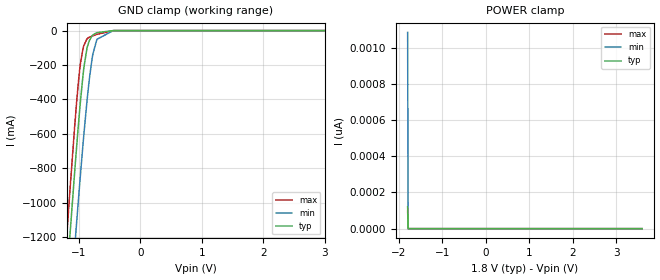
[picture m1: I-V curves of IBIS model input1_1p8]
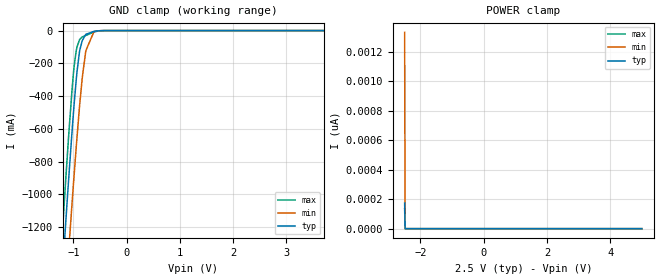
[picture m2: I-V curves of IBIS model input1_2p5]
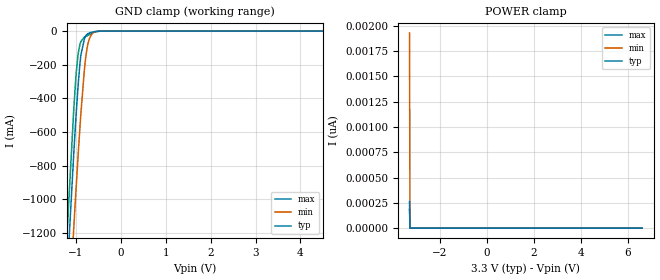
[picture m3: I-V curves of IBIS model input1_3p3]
| Texas Instruments Incorporated
| ADS93xx
| 2-Channel, 16-Bit 5/3 MSPS per channel
[IBIS Ver]   4.1
[File name]   ads93xx.ibs
[File Rev]   1.0
[Date]   28/03/2025
[Source]
| Texas Instruments Incorporated.
| Analog-eLab Design Center, HPA
| 12500 TI Blvd
| Dallas, TX -75243
[Notes]   Revision History:
| Rev 1.0: 28/03/2025
| - Initial version of the model
| - Model generated from simulations in SPECTRE
| - Model matched to SPICE simulation
| - C_comp although listed in numerical order of value are
|   obtained from varying PVT conditions. For PVT conditions for
|   each specific value refer the buffer description under
|   respective [Model]. IBIS model user is responsible for using
|   appropriate C_comp to simulate for Signal Integrity.
| - Warnings regarding combined Non-monotonicity of various models have been
|   reviewed and considered minor and can be ignored.
[Disclaimer]
| This model is designed as an aid for customers of Texas Instruments.
| TI and its licensors and suppliers make no warranties, either expressed
| or implied, with respect to this  model, including the warranties of
| merchantability or fitness for a particular purpose. The model is
| provided solely on an "as is" basis. The entire risk as to its quality
| and performance is with the customer.
[Copyright]
(C) Copyright 2025 Texas Instruments Incorporated.All rights reserved.
|   ADS9327, ADS9326
[Component]   ADS93xx
[Manufacturer]   TI
[Package]   |22 VQFN
|   typ   min   max
R_pkg   0.003   0.001   0.005
L_pkg   0.1nH   0.05nH   0.15nH
C_pkg   0.5pF   0.1pF   0.7pF
[Pin]  signal_name   model_name   R_pin   L_pin   C_pin
1   AINM_B   NC   NA   NA   NA
2   AINP_B   NC   NA   NA   NA
3   REF_CAP   NC   NA   NA   NA
4   REFM   NC   NA   NA   NA
5   AINM_A   NC   NA   NA   NA
6   AINP_A   NC   NA   NA   NA
7   AVDD   POWER   NA   NA   NA
8   GND   GND   NA   NA   NA
9   REFIO   NC   NA   NA   NA
10   CONVST   INPUT1   NA   NA   NA
11   CSZ   INPUT2   NA   NA   NA
12   SDI   INPUT2   NA   NA   NA
13   D3   OUTPUT   NA   NA   NA
14   D2   OUTPUT   NA   NA   NA
15   D1   OUTPUT   NA   NA   NA
16   D0   OUTPUT   NA   NA   NA
17   SCLK   INPUT2   NA   NA   NA
18   IOGND   GND   NA   NA   NA
19   IOVDD   POWER   NA   NA   NA
20   REF_SEL   INPUT3   NA   NA   NA
21   GND   GND   NA   NA   NA
22   VDD_1V8   POWER   NA   NA   NA
|   Model Selectors
[Model Selector] INPUT1
input1_1p8   1.8V   digital Input
input1_2p5   2.5V   digital Input
input1_3p3   3.3V   digital Input
[Model Selector] INPUT2
input2_1p8   1.8V   digital Input
input2_2p5   2.5V   digital Input
input2_3p3   3.3V   digital Input
[Model Selector] INPUT3
input3_1p8   1.8V   digital Input
input3_2p5   2.5V   digital Input
input3_3p3   3.3V   digital Input
[Model Selector] OUTPUT
output1_1p8   1.8V  digital 3-state
output1_2p5   2.5V  digital 3-state
output1_3p3   3.3V  digital 3-state
output1_1p8_0p5x   1.8V  digital 3-state
output1_2p5_0p5x   2.5V  digital 3-state
output1_3p3_0p5x   3.3V  digital 3-state
output1_1p8_2x   1.8V  digital 3-state
output1_2p5_2x   2.5V  digital 3-state
output1_3p3_2x   3.3V  digital 3-state
output1_1p8_1p5x   1.8V  digital 3-state
output1_2p5_1p5x   2.5V  digital 3-state
output1_3p3_1p5x   3.3V  digital 3-state
| Models and submodels in the file (21): input1_1p8 (Input), input1_2p5 (Input), input1_3p3 (Input), input2_1p8 (Input), input2_2p5 (Input), input2_3p3 (Input), input3_1p8 (Input), input3_2p5 (Input), input3_3p3 (Input), output1_1p8 (3-state), output1_2p5 (3-state), output1_3p3 (3-state), output1_1p8_0p5x (3-state), output1_2p5_0p5x (3-state), output1_3p3_0p5x (3-state), output1_1p8_2x (3-state), output1_2p5_2x (3-state), output1_3p3_2x (3-state), output1_1p8_1p5x (3-state), output1_2p5_1p5x (3-state), output1_3p3_1p5x (3-state)
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|   input1_1p8 Model
[Model]   input1_1p8
Model_type   Input
Vinl = 0.5
Vinh = 1.3
|   typ   min   max
C_comp   0.843pF   0.797pF   0.882pF
[Voltage Range]   1.8   1.65   1.95
[Temperature Range]   27   125   -40
[Power Clamp Reference]   1.8   1.65   1.95
[GND Clamp Reference]   0   0   0
[GND Clamp]
|   Voltage   I(typ)   I(min)   I(max)
-1.8V     -4.331A    -4.221A    -4.398A
-1.201V   -1.449A    -1.88A     -1.194A
-1.147V   -1.182A    -1.619A    -920.4mA
-1.071V   -819.9mA   -1.262A    -555.7mA
-1.044V   -696.1mA   -1.137A    -435.4mA
-979.2mV  -419mA     -846.7mA   -195.6mA
-919.8mV  -211.4mA   -597mA     -85.4mA
-865.8mV  -95.01mA   -392.5mA   -46.28mA
-774mV    -24.87mA   -135.4mA   -30.61mA
-709.2mV  -12.08mA   -51mA      -22.01mA
-444.6mV  -241.7uA   -227.8uA   -354uA
3.6V      0A         0A         0A
[POWER Clamp]
|   Voltage   I(typ)   I(min)   I(max)
-1.8V     121.1pA    1.084nA    96.11pA
-1.789V   0A         0A         0A
-1.784V   0A         0A         0A
3.6V      0A         0A         0A
|   input1_2p5 Model
[Model]   input1_2p5
Model_type   Input
Vinl = 0.5
Vinh = 2
|   typ   min   max
C_comp   0.794pF   0.748pF   0.831pF
[Voltage Range]   2.5   2.4   2.6
[Temperature Range]   27   125   -40
[Power Clamp Reference]   2.5   2.4   2.6
[GND Clamp Reference]   0   0   0
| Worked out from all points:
|   GND clamp passes 1 mA (typ) near -0.51 V on its own axis
[GND Clamp]
|   Voltage   I(typ)   I(min)   I(max)
-2.5V     -6.194A    -5.986A    -6.426A
-1.21V    -1.496A    -1.925A    -1.243A
-1.143V   -1.162A    -1.599A    -899.9mA
-1.083V   -873.7mA   -1.315A    -609mA
-1V       -504mA     -938.2mA   -261.8mA
-947.5mV  -300.2mA   -710.9mA   -122.9mA
-880mV    -117.7mA   -443.5mA   -52.77mA
-835mV    -61.28mA   -290.5mA   -38.71mA
-767.5mV  -22.75mA   -123.3mA   -29.8mA
-617.5mV  -4.872mA   -8.587mA   -9.146mA
-520mV    -1.284mA   -1.107mA   -2.265mA
5V        0A         0A         0A
[POWER Clamp]
|   Voltage   I(typ)   I(min)   I(max)
-2.5V     173.2pA    1.33nA     134pA
-2.485V   0A         0A         0A
-2.478V   0A         0A         0A
5V        0A         0A         0A
|   input1_3p3 Model
[Model]   input1_3p3
Model_type   Input
Vinl = 0.5
Vinh = 2.8
|   typ   min   max
C_comp   0.761pF   0.724pF   0.797pF
[Voltage Range]   3.3   3   3.5
[Temperature Range]   27   125   -40
[Power Clamp Reference]   3.3   3   3.5
[GND Clamp Reference]   0   0   0
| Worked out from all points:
|   GND clamp passes 1 mA (typ) near -0.50 V on its own axis
[GND Clamp]
|   Voltage   I(typ)   I(min)   I(max)
-3.3V     -8.304A    -7.999A    -8.643A
-1.241V   -1.651A    -2.076A    -1.403A
-1.053V   -735.6mA   -1.177A    -473.3mA
-993.3mV  -476.1mA   -908.6mA   -239.1mA
-953.7mV  -322.2mA   -737.1mA   -134.3mA
-894.3mV  -146.2mA   -497.1mA   -62.78mA
-795.3mV  -34.72mA   -181.3mA   -33.23mA
-755.7mV  -19.61mA   -103.6mA   -28.31mA
-716.1mV  -12.9mA    -56.72mA   -23.09mA
-617.1mV  -4.851mA   -8.509mA   -9.105mA
-458.7mV  -350uA     -312.3uA   -541uA
6.6V      0A         0A         0A
[POWER Clamp]
|   Voltage   I(typ)   I(min)   I(max)
-3.3V     263.6pA    1.931nA    187.9pA
-3.28V    0A         0A         0A
-3.27V    0A         0A         0A
6.6V      0A         0A         0A
